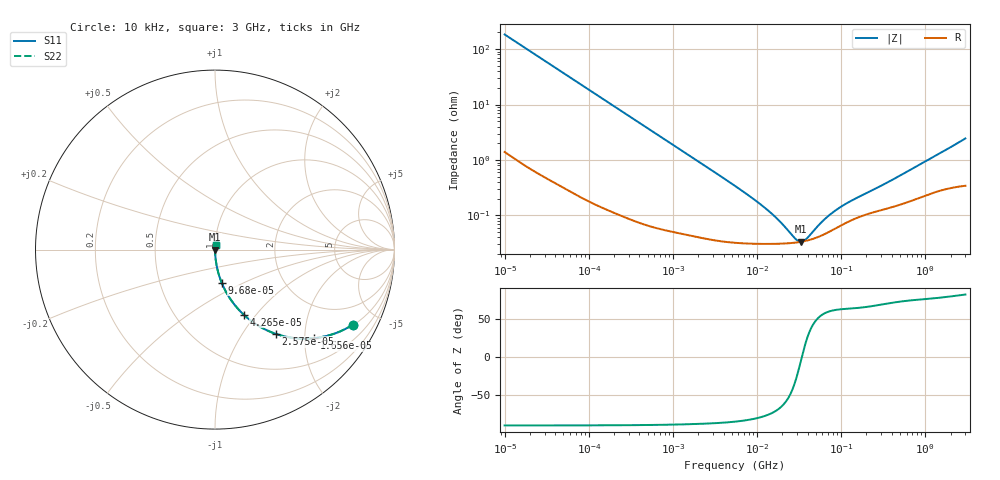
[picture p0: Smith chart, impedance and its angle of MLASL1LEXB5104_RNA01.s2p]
! MLASL1LEXB5104_RNA01  S-PARAMETER MODEL  ( Standard Model )
! Model Generated by TAIYO YUDEN Corporation (http://www.ty-top.com)
! Version 2.0
! TAIYO YUDEN Control No. 230320
! Copyright(c) 2015 TAIYO YUDEN CO.,LTD. All Rights Reserved.
! Product Description (link to TY-COMPAS)
! https://ds.yuden.co.jp/TYCOMPAS/or/detail?pn=MLASL1LEXB5104KRNA01&u=M
! Products Name : Multilayer Ceramic Capacitors
! Characteristics :
!  Capacitance : 0.1 [uF] , Rated Voltage : 10 [V] , TCC : X5R
!  Case Size : 1.0 x 0.5 / 0.039 x 0.02 [mm/inch] , Thickness : 0.18 / 0.007 [mm/inch]
!  (Conditions: Temperature = 25 [degC] , DC Bias Voltage = 0 [V])
! External Node Assignments :
!  1  o---| |---o  2
! GND o---------o GND
! Frequency Range : 10kHz  -  3GHz  [ 401 STEP ]
# MHZ S RI R 50
! Freq[MHz].  S11 Real  S11 Imag  S21 Real  S21 Imag  S12 Real  S12 Imag  S22 Real  S22 Imag
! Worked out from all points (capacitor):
!   401 points, 10 kHz to 3 GHz, reference 50 ohm
!   read as one part in series: C = 86.6 nF near 10.65 kHz
!   lowest |Z| = 33.5 mohm at 33.04 MHz (marker M1)
!   series resonance near 34.1 MHz, so ESL is about 250 pH
!   S11 on the Smith chart (normalised r, x): 10 kHz: 1.03, -3.67; 16.56 kHz: 1.02, -2.22; 25.75 kHz: 1.01, -1.43; 42.65 kHz: 1.01, -0.87; 96.8 kHz: 1.00, -0.38; 3 GHz: 1.01, +0.05
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0.01  0.7695 -0.4174  0.2305 0.4174  0.2305 0.4174  0.7695 -0.4174
0.012083  0.6968 -0.4559  0.3032 0.4559  0.3032 0.4559  0.6968 -0.4559
0.016561  0.5521 -0.4935  0.4479 0.4935  0.4479 0.4935  0.5521 -0.4935
0.02575  0.34 -0.4699  0.66 0.4699  0.66 0.4699  0.34 -0.4699
0.042645  0.1601 -0.3626  0.8399 0.3626  0.8399 0.3626  0.1601 -0.3626
0.058452  0.0932 -0.2863  0.9068 0.2863  0.9068 0.2863  0.0932 -0.2863
0.082683  0.0496 -0.2126  0.9504 0.2126  0.9504 0.2126  0.0496 -0.2126
0.096801  0.0371 -0.1842  0.9629 0.1842  0.9629 0.1842  0.0371 -0.1842
0.226771  0.00771 -0.0814  0.9923 0.0814  0.9923 0.0814  0.00771 -0.0814
0.683653  0.00132 -0.0274  0.9987 0.0274  0.9987 0.0274  0.00132 -0.0274
5.477226  0.000332 -0.00339  0.9997 0.00339  0.9997 0.00339  0.000332 -0.00339
13.66633  0.000307 -0.00117  0.9997 0.00117  0.9997 0.00117  0.000307 -0.00117
18.73182  0.000309 -0.000714  0.9997 0.000714  0.9997 0.000714  0.000309 -0.000714
28.22191  0.000322 -0.000214  0.9997 0.000214  0.9997 0.000214  0.000322 -0.000214
33.04079  0.000333 -3.53e-05  0.9997 3.53e-05  0.9997 3.53e-05  0.000333 -3.53e-05
37.4819  0.000346 0.000106  0.9997 -0.000106  0.9997 -0.000106  0.000346 0.000106
45.28751  0.000373 0.00032  0.9996 -0.00032  0.9996 -0.00032  0.000373 0.00032
64.06182  0.000462 0.000726  0.9995 -0.000726  0.9995 -0.000726  0.000462 0.000726
93.52181  0.000626 0.00119  0.9994 -0.00119  0.9994 -0.00119  0.000626 0.00119
136.5295  0.000836 0.00169  0.9992 -0.00169  0.9992 -0.00169  0.000836 0.00169
374.4521  0.00138 0.00386  0.9986 -0.00386  0.9986 -0.00386  0.00138 0.00386
3000  0.00399 0.024  0.996 -0.024  0.996 -0.024  0.00399 0.024
